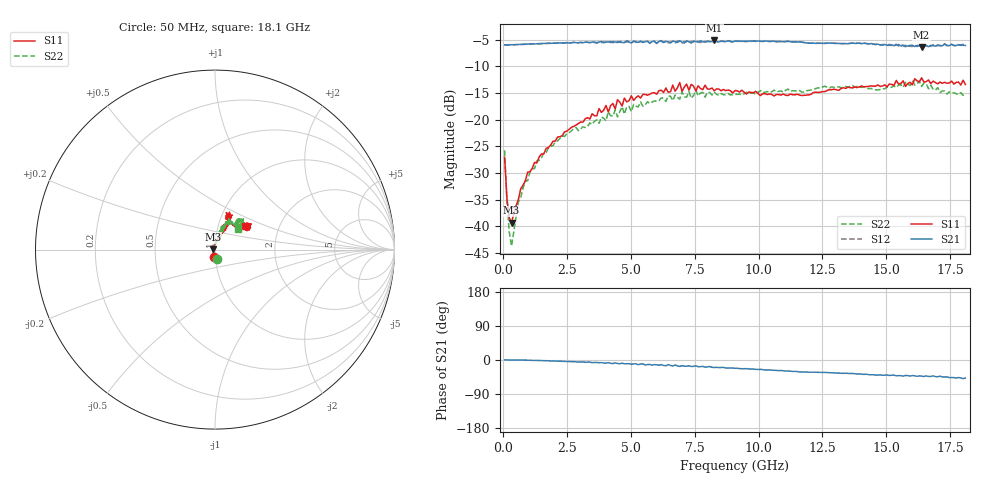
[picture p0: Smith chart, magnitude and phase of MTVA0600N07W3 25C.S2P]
! Network Analyzer HP8720D.06.14 Serial No. US36140669
!  8 Jul 2005  12:20:07
! Frequency  S11  S21  S12  S22
# HZ  S  DB R 50
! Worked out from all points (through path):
!   201 points, 50 MHz to 18.1 GHz, reference 50 ohm
!   highest |S21| = -5.12 dB at 8.263 GHz (marker M1); lowest = -6.3 dB at 16.39 GHz (marker M2)
!   group delay of S21, straight-line fit = 7.84 ps
!   lowest |S11| = -39.4 dB at 320.8 MHz (marker M3), VSWR 1.02, Z = 49 + j0.211 ohm
!   |S11| at or under -10 dB: start of sweep to end of sweep
!   |S22| runs from -43.7 to -12.6 dB; largest |S21 - S12| = 0.028
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5e7  -27.04 -99.1  -5.93 0.2  -5.94 0.4  -25.75 -74.6
1.4025e8  -34.73 -122.4  -5.99 0.1  -5.99 0.1  -35.30 -107.0
2.305e8  -38.37 -154.1  -5.95 0.2  -5.95 0.1  -41.00 -138.3
3.2075e8  -39.36 168.5  -5.91 0.2  -5.93 0.3  -43.75 167.2
5.915e8  -34.96 114.5  -5.87 0.1  -5.90 0.0  -35.40 107.2
1.04275e9  -29.78 92.9  -5.77 -0.7  -5.79 -0.7  -29.82 84.8
2.12575e9  -23.25 70.9  -5.61 -3.1  -5.61 -3.0  -23.99 74.3
3.1185e9  -20.46 68.8  -5.52 -4.9  -5.56 -5.3  -21.34 74.8
4.021e9  -17.33 67.2  -5.41 -8.3  -5.45 -7.2  -20.23 70.9
4.11125e9  -18.57 67.1  -5.39 -6.9  -5.48 -8.5  -18.52 70.6
4.47225e9  -16.25 61.9  -5.51 -9.2  -5.32 -8.2  -19.48 75.4
4.65275e9  -17.43 62.4  -5.51 -8.4  -5.35 -10.0  -17.55 75.1
4.743e9  -15.95 65.5  -5.53 -9.9  -5.44 -8.9  -18.95 71.4
6.09675e9  -14.54 64.9  -5.32 -13.9  -5.24 -13.7  -16.40 67.2
6.909e9  -13.02 68.9  -5.17 -17.0  -5.28 -15.1  -16.15 61.8
6.99925e9  -14.67 69.0  -5.44 -14.8  -5.60 -16.8  -14.76 63.2
8.26275e9  -14.56 68.5  -5.12 -19.8  -5.33 -20.4  -14.82 57.0
9.075e9  -14.52 65.9  -5.25 -21.6  -5.22 -21.8  -15.21 55.8
1.21435e10  -14.90 49.2  -5.62 -32.1  -5.57 -32.3  -14.31 51.8
1.512175e10  -13.28 31.6  -6.04 -40.8  -5.84 -40.5  -13.95 52.6
1.638525e10  -12.13 35.4  -6.32 -42.7  -6.06 -41.9  -13.76 46.2
1.81e10  -13.38 38.4  -6.06 -47.8  -6.25 -48.3  -15.30 41.5
